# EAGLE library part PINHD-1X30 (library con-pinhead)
PIN HEADER
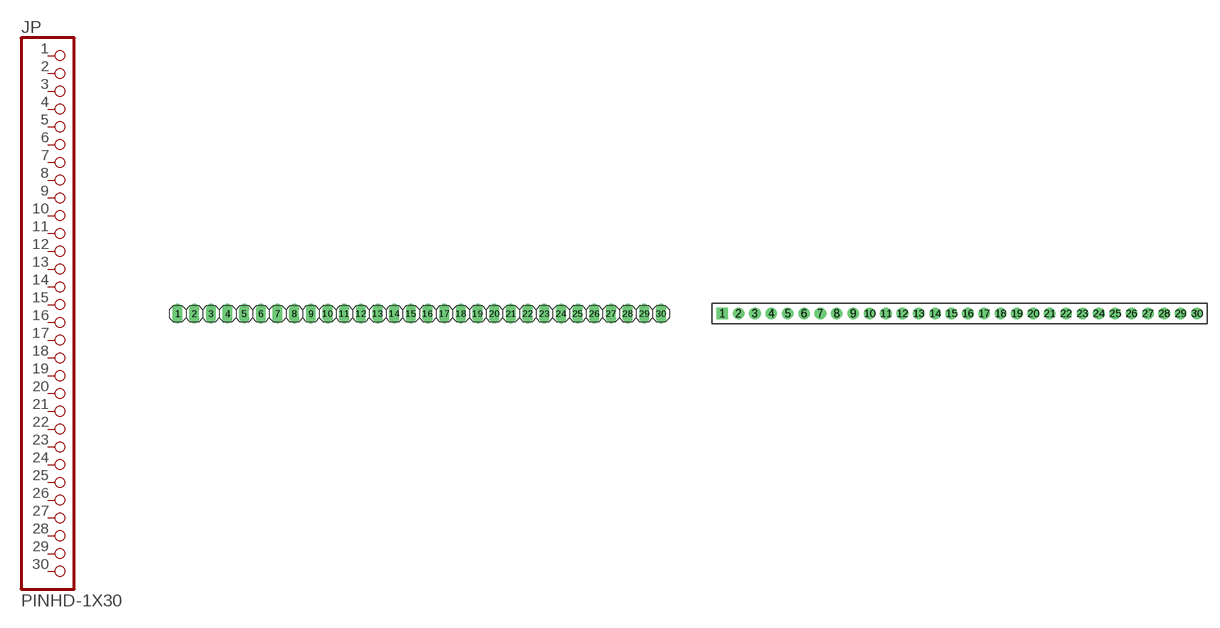
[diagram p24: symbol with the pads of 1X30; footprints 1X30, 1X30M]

Designator prefix JP

## PINHD-1X30_2.54  [1X30]
1  1  pas
2  2  pas
3  3  pas
4  4  pas
5  5  pas
6  6  pas
7  7  pas
8  8  pas
9  9  pas
10  10  pas
11  11  pas
12  12  pas
13  13  pas
14  14  pas
15  15  pas
16  16  pas
17  17  pas
18  18  pas
19  19  pas
20  20  pas
21  21  pas
22  22  pas
23  23  pas
24  24  pas
25  25  pas
26  26  pas
27  27  pas
28  28  pas
29  29  pas
30  30  pas

## PINHD-1X30_2.00  [1X30M]
Pads as for 1X30

## PINHD-1X30_2.54-90°  [1X30/90]
Pads as for 1X30

## PINHD-1X30_2.54-SMD  [1X30SMD]
Pads as for 1X30

## PINHD-1X30_2.54-SMD-90°  [1X30SMD/90]
Pads as for 1X30

## Footprint 1X30 (pad centres in mm)
PIN HEADER - 2.54
drill 1.016 long: 1 -36.83,0; 2 -34.29,0; 3 -31.75,0; 4 -29.21,0; 5 -26.67,0; 6 -24.13,0; 7 -21.59,0; 8 -19.05,0; 9 -16.51,0; 10 -13.97,0; 11 -11.43,0; 12 -8.89,0; 13 -6.35,0; 14 -3.81,0; 15 -1.27,0; 16 1.27,0; 17 3.81,0; 18 6.35,0; 19 8.89,0; 20 11.43,0; 21 13.97,0; 22 16.51,0; 23 19.05,0; 24 21.59,0; 25 24.13,0; 26 26.67,0; 27 29.21,0; 28 31.75,0; 29 34.29,0; 30 36.83,0

## Footprint 1X30M (pad centres in mm)
PIN HEADER - 2
drill 0.914 square: 1 -29,0
drill 0.914: 2 -27,0; 3 -25,0; 4 -23,0; 5 -21,0; 6 -19,0; 7 -17,0; 8 -15,0; 9 -13,0; 10 -11,0; 11 -9,0; 12 -7,0; 13 -5,0; 14 -3,0; 15 -1,0; 16 1,0; 17 3,0; 18 5,0; 19 7,0; 20 9,0; 21 11,0; 22 13,0; 23 15,0; 24 17,0; 25 19,0; 26 21,0; 27 23,0; 28 25,0; 29 27,0; 30 29,0

## Footprint 1X30/90 (pad centres in mm)
PIN HEADER - 2.54 90°
drill 1.016 long: 1 -24.13,-3.81; 2 -21.59,-3.81; 3 -19.05,-3.81; 4 -16.51,-3.81; 5 -13.97,-3.81; 6 -11.43,-3.81; 7 -8.89,-3.81; 8 -6.35,-3.81; 9 -3.81,-3.81; 10 -1.27,-3.81; 11 1.27,-3.81; 12 3.81,-3.81; 13 6.35,-3.81; 14 8.89,-3.81; 15 11.43,-3.81; 16 13.97,-3.81; 17 16.51,-3.81; 18 19.05,-3.81; 19 21.59,-3.81; 20 24.13,-3.81; 21 26.67,-3.81; 22 29.21,-3.81; 23 31.75,-3.81; 24 34.29,-3.81; 25 36.83,-3.81; 26 39.37,-3.81; 27 41.91,-3.81; 28 44.45,-3.81; 29 46.99,-3.81; 30 49.53,-3.81

## Footprint 1X30SMD (pad centres in mm)
PIN HEADER - 2.54 SMD
smd 1.016 x 3.302: 1 -1.27,1.27; 2 1.27,-1.27; 3 3.81,1.27; 4 6.35,-1.27; 5 8.89,1.27; 6 11.43,-1.27; 7 13.97,1.27; 8 16.51,-1.27; 9 19.05,1.27; 10 21.59,-1.27; 11 24.13,1.27; 12 26.67,-1.27; 13 29.21,1.27; 14 31.75,-1.27; 15 34.29,1.27; 16 36.83,-1.27; 17 39.37,1.27; 18 41.91,-1.27; 19 44.45,1.27; 20 46.99,-1.27; 21 49.53,1.27; 22 52.07,-1.27; 23 54.61,1.27; 24 57.15,-1.27; 25 59.69,1.27; 26 62.23,-1.27; 27 64.77,1.27; 28 67.31,-1.27; 29 69.85,1.27; 30 72.39,-1.27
